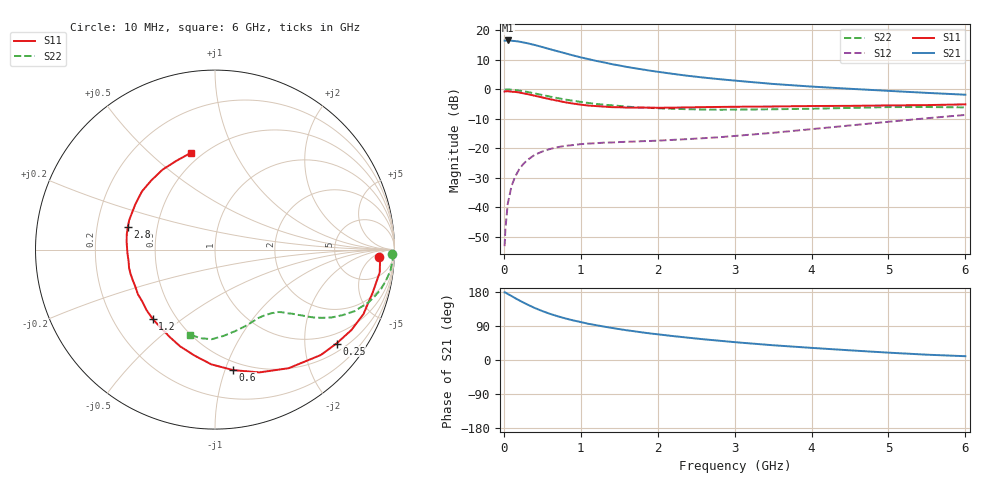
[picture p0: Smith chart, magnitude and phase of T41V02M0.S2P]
! Infineon Technologies  Discrete & RF Semiconductors
! BFR182T
! Si NPN RF Bipolar Junction Transistor in SC75
! VCE = 1 V  IC = 2 mA
! Common Emitter S-Parameters:  October  1999
# GHz  S  MA  R  50
!  f  S11  S21  S12  S22
! GHz  MAG  ANG  MAG  ANG  MAG  ANG  MAG  ANG
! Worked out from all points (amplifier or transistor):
!   36 points, 10 MHz to 6 GHz, reference 50 ohm
!   highest |S21| = 16.5 dB at 50 MHz (marker M1)
!   |S21| within 3 dB of that: start of sweep to 605.8 MHz
!   unconditionally stable (mu >= 1): 1.884 GHz to 4.666 GHz
!   at 250 MHz: K = 0.16, MSG = 20.7 dB, |S12| = -25.4 dB
!   at 1.4 GHz: K = 0.80, MSG = 13.3 dB, |S12| = -18.0 dB
!   at 6 GHz: K = 0.89, MSG = 3.4 dB, |S12| = -8.7 dB
!   S11 on the Smith chart (normalised r, x): 10 MHz: 18, -9; 250 MHz: 0.71, -2.77; 600 MHz: 0.43, -1.07; 1.2 GHz: 0.37, -0.39; 2.8 GHz: 0.34, +0.11; 6 GHz: 0.44, +0.68
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0.01  0.915 -2.7  6.683 178.4  0.0022 85.8  0.9888 -1.5
0.02  0.9214 -1.8  6.649 178.1  0.0042 90.0  0.9865 -1.4
0.05  0.9264 -7.9  6.713 174.3  0.0113 88.0  0.9912 -3.5
0.1  0.9105 -15.3  6.628 168.9  0.023 82.4  0.9842 -6.9
0.15  0.9018 -23.5  6.549 162.9  0.0337 76.1  0.9684 -10.2
0.25  0.8556 -37.7  6.234 152.1  0.0536 68.8  0.928 -16.2
0.3  0.8321 -44.9  6.04 147.0  0.0625 65.6  0.9051 -18.9
0.4  0.7777 -58.2  5.635 137.4  0.0774 59.3  0.8514 -23.7
0.5  0.7273 -70.2  5.196 129.2  0.0882 54.2  0.7991 -27.2
0.6  0.6786 -81.5  4.775 121.8  0.0974 50.1  0.7519 -30.2
0.7  0.6399 -91.8  4.401 115.4  0.1047 46.3  0.7077 -32.5
0.8  0.6015 -100.9  4.066 109.7  0.1101 43.7  0.6697 -34.4
0.9  0.5727 -109.9  3.744 104.6  0.1135 41.7  0.6367 -35.9
1.1  0.5294 -125.1  3.244 95.5  0.1204 39.0  0.5863 -38.3
1.2  0.5191 -132.0  3.027 91.9  0.1221 37.9  0.5645 -39.4
1.6  0.4892 -155.4  2.39 78.4  0.129 37.1  0.5082 -43.3
2.2  0.4886 -178.2  1.823 63.1  0.1391 40.7  0.468 -50.1
2.8  0.502 165.4  1.484 50.9  0.1541 45.7  0.4506 -58.4
3.5  0.5107 150.5  1.231 38.9  0.1832 50.9  0.4588 -68.5
4.5  0.5238 132.8  1.019 25.5  0.2439 53.9  0.4829 -84.2
5.5  0.5396 113.4  0.869 14.0  0.3234 51.5  0.5004 -99.2
6  0.5552 104.1  0.809 10.0  0.3677 48.4  0.4935 -106.1
